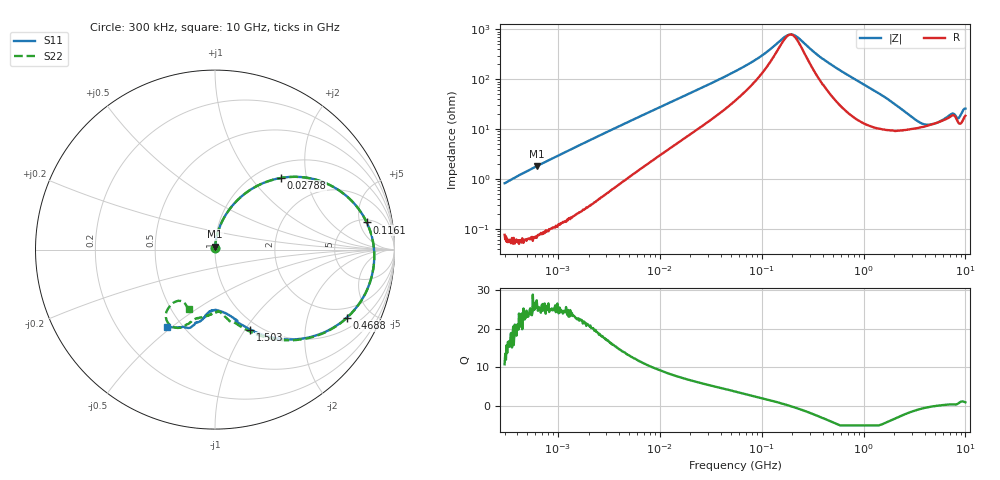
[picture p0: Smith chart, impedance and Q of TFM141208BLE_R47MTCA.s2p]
! S-Parameter Data Generated by TDK Corporation
! Copyright(C) 2026 TDK Corporation.
! All Rights Reserved.
! TDK P/N: TFM141208BLE-R47MTCA (SMD / SMT Inductor (Coil))
! Property: L=0.47uH at 1MHz
! Size(LxWxT): 1.4x1.2x0.8mm
! Model Type: s2p (Touchstone File Format Version 1.0)
! Frequency: DC=Yes Start=0.3MHz Stop=10000MHz 802points Log-sweep
! Model Generated on Feb. 24, 2026
! Terms and conditions regarding TDK Simulation Models:
! 1)This simulation model is being provided solely for informational
!  purposes. Please refer to the specifications of the products in
!  terms of detailed characteristics of such products.
! 2)In no event shall TDK Corporation of any of its subsidiaries be
!  liable for any loss or damage arising, directly or indirectly,
!  from any information contained in this simulation model, including,
!  but not limited to loss or damages arising from any inaccuracies,
!  omissions or errors in connection with such information.
! 3)Any and all copyrights on this simulation model are owned by
!  TDK Corporation.  Duplication or redistribution of this simulation
!  model without prior written permission from TDK Corporation
!  is prohibited.
! 4)This simulation model is subject to any modification or change
!  without any prior notice.
! 5)Neither TDK Corporation nor any of its subsidiaries shall make any
!  warranty, express or implied, including but not limited to the
!  correctness, implied warranties of merchantability and fitness for
!  a particular purpose with respect to this simulation models.
! 6)The use of this simulation model shall be deemed to have consented
!  to the terms and conditions hereof.
! Port Assignments:
!  1 ---@@@--- 2
! Applicable Conditions:
!  Temperature = 25 degC
!  DC Bias Current = 0 A
!  Small Signal Operation
# Hz S MA R 50
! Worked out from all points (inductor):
!   801 points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, 300 kHz to 10 GHz, reference 50 ohm
!   read as one part in series: L = 450 nH near 318.3 kHz
!   highest Q = 25.7 at 619.1 kHz (marker M1), where L = 462 nH
!   self-resonance near 191.5 MHz
!   S11 on the Smith chart (normalised r, x): 300 kHz: 1.00, +0.01; 27.88 MHz: 1.26, +1.43; 116.1 MHz: 5.60, +6.47; 468.8 MHz: 1.47, -3.52; 1.503 GHz: 0.90, -1.06; 10 GHz: 0.42, -0.48
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300000  0.006558 84.5  0.9992 -0.6  0.9993 -0.5  0.006614 81.2
619123  0.0171 86.7  0.9991 -1.1  0.9992 -1.1  0.01698 86.7
1713600  0.04917 84.6  0.9965 -2.9  0.9966 -2.9  0.04918 84.5
9671944  0.2502 69.4  0.9419 -14.5  0.942 -14.5  0.2501 69.4
1.649435e7  0.3839 59.6  0.8725 -22.5  0.8724 -22.5  0.3839 59.6
2.78833e7  0.5437 47.3  0.7497 -32.7  0.7497 -32.7  0.5437 47.3
5.477226e7  0.7354 29.2  0.514 -45.9  0.5141 -45.9  0.7354 29.2
1.161426e8  0.8589 10.2  0.2315 -48.2  0.2315 -48.2  0.8588 10.1
1.6757e8  0.8841 1.3  0.126 -23.5  0.1261 -23.5  0.8842 1.2
1.945824e8  0.8881 -2.4  0.1119 0.9  0.112 0.9  0.8883 -2.5
2.257919e8  0.8885 -6.2  0.1279 25.2  0.1279 25.2  0.8888 -6.3
3.126428e8  0.8756 -15.1  0.2288 48.1  0.2289 48.1  0.8759 -15.2
4.687561e8  0.8256 -27.4  0.3961 48.4  0.3961 48.4  0.8264 -27.6
8.299813e8  0.6782 -47.4  0.6348 33.8  0.6349 33.7  0.6813 -47.6
1.50342e9  0.4869 -66.2  0.7913 14.2  0.7915 14.1  0.4935 -67.2
1.767019e9  0.4434 -70.6  0.8162 8.8  0.8163 8.8  0.4486 -72.0
2.659614e9  0.3652 -79.2  0.8462 -4.4  0.8464 -4.5  0.3637 -83.1
4.049484e9  0.3396 -91.9  0.8341 -18.3  0.8344 -18.3  0.3508 -90.2
6.899057e9  0.4191 -104.2  0.7453 -40.4  0.7451 -40.4  0.4189 -108.1
8.09931e9  0.4551 -107.4  0.7083 -44.8  0.7092 -44.9  0.4908 -119.3
8.770142e9  0.4633 -110.3  0.7512 -48.1  0.7514 -48.3  0.4382 -128.1
1e10  0.5041 -121.7  0.6973 -57.9  0.6974 -58.0  0.3624 -114.0
